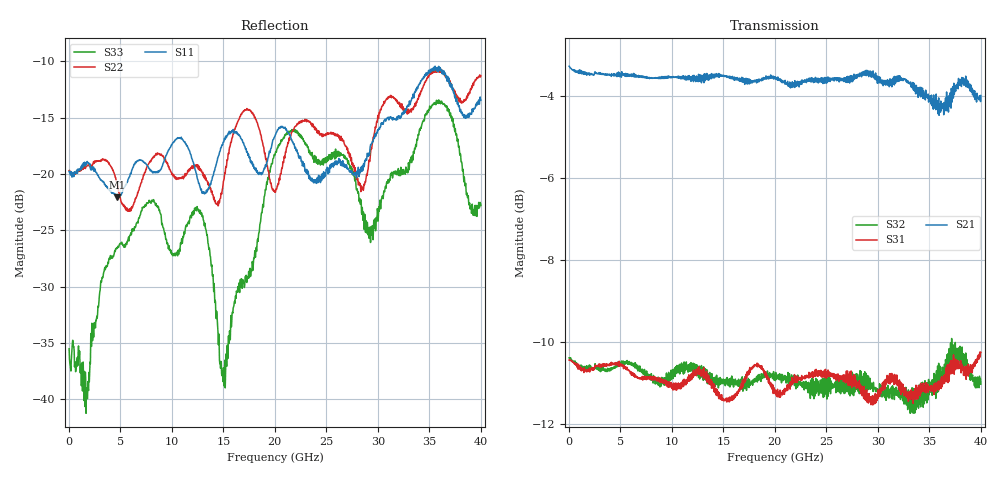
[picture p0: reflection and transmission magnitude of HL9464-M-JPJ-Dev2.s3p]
! 3/9/2020 2:48:47 PM
! H:\PRODUCTION_DATA\TEMP_S3P.S3P
! CHANNEL.1
! TR.MEASUREMENT
! CORRECTED.DATA
# GHZ S RI R 50.0
! FREQ.GHZ  S11RE  S11IM  S12RE  S12IM  S13RE  S13IM
!  S21RE  S21IM  S22RE  S22IM  S23RE  S23IM
!  S31RE  S31IM  S32RE  S32IM  S33RE  S33IM
!; PortSelection: Port_123
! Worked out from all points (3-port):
!   1143 points, 35 MHz to 40.01 GHz, reference 50 ohm
!   strongest paths, dB at 35 MHz, 10.01 GHz, 20.02 GHz, 30.03 GHz, 40.01 GHz:
!     S21: -3.3, -3.5, -3.6, -3.5, -4.0
!     S31: -10.4, -11.1, -11.2, -11.4, -10.3
!     S32: -10.4, -10.9, -10.8, -11.2, -11.0
!   lowest |S11| = -22.1 dB at 4.725 GHz (marker M1), VSWR 1.17, Z = 44.1 + j4.48 ohm
!   |S11| at or under -10 dB: start of sweep to end of sweep
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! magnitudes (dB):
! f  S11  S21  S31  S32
! 35 MHz  -19.8  -3.3  -10.4  -10.4
! 1.75 GHz  -18.9  -3.5  -10.7  -10.6
! 4.725 GHz  -22.1  -3.5  -10.6  -10.6
! 12.6 GHz  -20.8  -3.5  -10.8  -10.9
! 15.05 GHz  -17.2  -3.5  -11.4  -11.0
! 17.43 GHz  -18.2  -3.7  -10.7  -10.9
! 20.02 GHz  -16.6  -3.6  -11.2  -10.8
! 29.36 GHz  -17.3  -3.6  -11.4  -11.1
! 36.09 GHz  -10.7  -4.4  -10.9  -11.1
! 40.01 GHz  -13.4  -4.0  -10.3  -11.0
